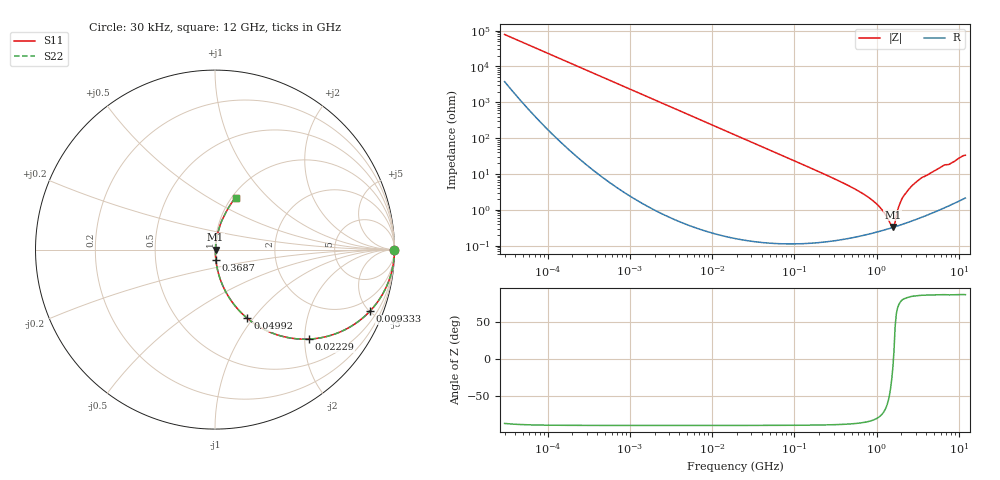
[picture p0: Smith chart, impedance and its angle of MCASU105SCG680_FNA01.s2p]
! MCASU105SCG680_FNA01  S-PARAMETER MODEL  ( General Type )
! Model Generated by TAIYO YUDEN Corporation (http://www.ty-top.com)
! Version 1.0
! TAIYO YUDEN Control No. 130207
! Copyright(c) 2013 TAIYO YUDEN CO.,LTD. All Rights Reserved.
! Product Description (link to TY-COMPAS)
! https://ds.yuden.co.jp/TYCOMPAS/or/detail?pn=MCASU105SCG680JFNA01&u=M
! Products Name : Multilayer Ceramic Capacitors
! Characteristics :
!  Capacitance : 68 pF , Rated Voltage : 50V , TCC : CG / C0G
!  Case Size : 1.0 x 0.5 / 0.039 x 0.02 [mm/inch] , Thickness : 0.5 / 0.02 [mm/inch]
!  (Conditions: Temperature = 25 degC , DC Bias Current/Voltage = 0A / 0V)
! External Node Assignments :
!  1  o---| |---o  2
! GND o---------o GND
! Frequency Range : 30000Hz  -  12GHz  [ 401 STEP ]
# MHz S RI R 50
! Freq[MHz].  S11 Real  S11 Imag  S21 Real  S21 Imag  S12 Real  S12 Imag  S22 Real  S22 Imag
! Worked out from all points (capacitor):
!   401 points, 30 kHz to 12 GHz, reference 50 ohm
!   read as one part in series: C = 68 pF near 32 kHz
!   lowest |Z| = 331 mohm at 1.573 GHz (marker M1)
!   series resonance near 1.602 GHz, so ESL is about 150 pH
!   S11 on the Smith chart (normalised r, x): 30 kHz: open; 9.333 MHz: 1.00, -5.01; 22.29 MHz: 1.00, -2.10; 49.92 MHz: 1.00, -0.94; 368.7 MHz: 1.00, -0.12; 12 GHz: 1.04, +0.66
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0.03  0.9999 -0.00128  6.34e-05 0.00128  6.34e-05 0.00128  0.9999 -0.00128
0.260295  0.9998 -0.0111  0.000152 0.0111  0.000152 0.0111  0.9998 -0.0111
2.258455  0.9907 -0.0956  0.00931 0.0956  0.00931 0.0956  0.9907 -0.0956
5.223303  0.9523 -0.2126  0.0477 0.2126  0.0477 0.2126  0.9523 -0.2126
9.333359  0.8624 -0.344  0.1376 0.344  0.1376 0.344  0.8624 -0.344
18.97367  0.603 -0.4886  0.397 0.4886  0.397 0.4886  0.603 -0.4886
22.29344  0.5239 -0.4987  0.4761 0.4987  0.4761 0.4987  0.5239 -0.4987
49.92358  0.1804 -0.3832  0.8196 0.3832  0.8196 0.3832  0.1804 -0.3832
83.63502  0.0731 -0.2583  0.9269 0.2583  0.9269 0.2583  0.0731 -0.2583
164.6252  0.0205 -0.1376  0.9795 0.1376  0.9795 0.1376  0.0205 -0.1376
368.6592  0.00505 -0.0598  0.995 0.0598  0.995 0.0598  0.00505 -0.0598
909.4299  0.00256 -0.0175  0.9974 0.0175  0.9974 0.0175  0.00256 -0.0175
1177.092  0.00273 -0.00928  0.9973 0.00928  0.9973 0.00928  0.00273 -0.00928
1428.372  0.00302 -0.00356  0.997 0.00356  0.997 0.00356  0.00302 -0.00356
1573.464  0.00322 -0.000717  0.9968 0.000717  0.9968 0.000717  0.00322 -0.000717
1678.29  0.00338 0.00313  0.9966 -0.00313  0.9966 -0.00313  0.00338 0.00313
1848.769  0.00375 0.0112  0.9963 -0.0112  0.9963 -0.0112  0.00375 0.0112
2036.564  0.0043 0.0201  0.9957 -0.0201  0.9957 -0.0201  0.0043 0.0201
2722.352  0.00719 0.0475  0.9928 -0.0475  0.9928 -0.0475  0.00719 0.0475
3411.775  0.0113 0.0728  0.9887 -0.0728  0.9887 -0.0728  0.0113 0.0728
6296.196  0.0362 0.1571  0.9638 -0.1571  0.9638 -0.1571  0.0362 0.1571
12000  0.1144 0.2878  0.8856 -0.2878  0.8856 -0.2878  0.1144 0.2878
